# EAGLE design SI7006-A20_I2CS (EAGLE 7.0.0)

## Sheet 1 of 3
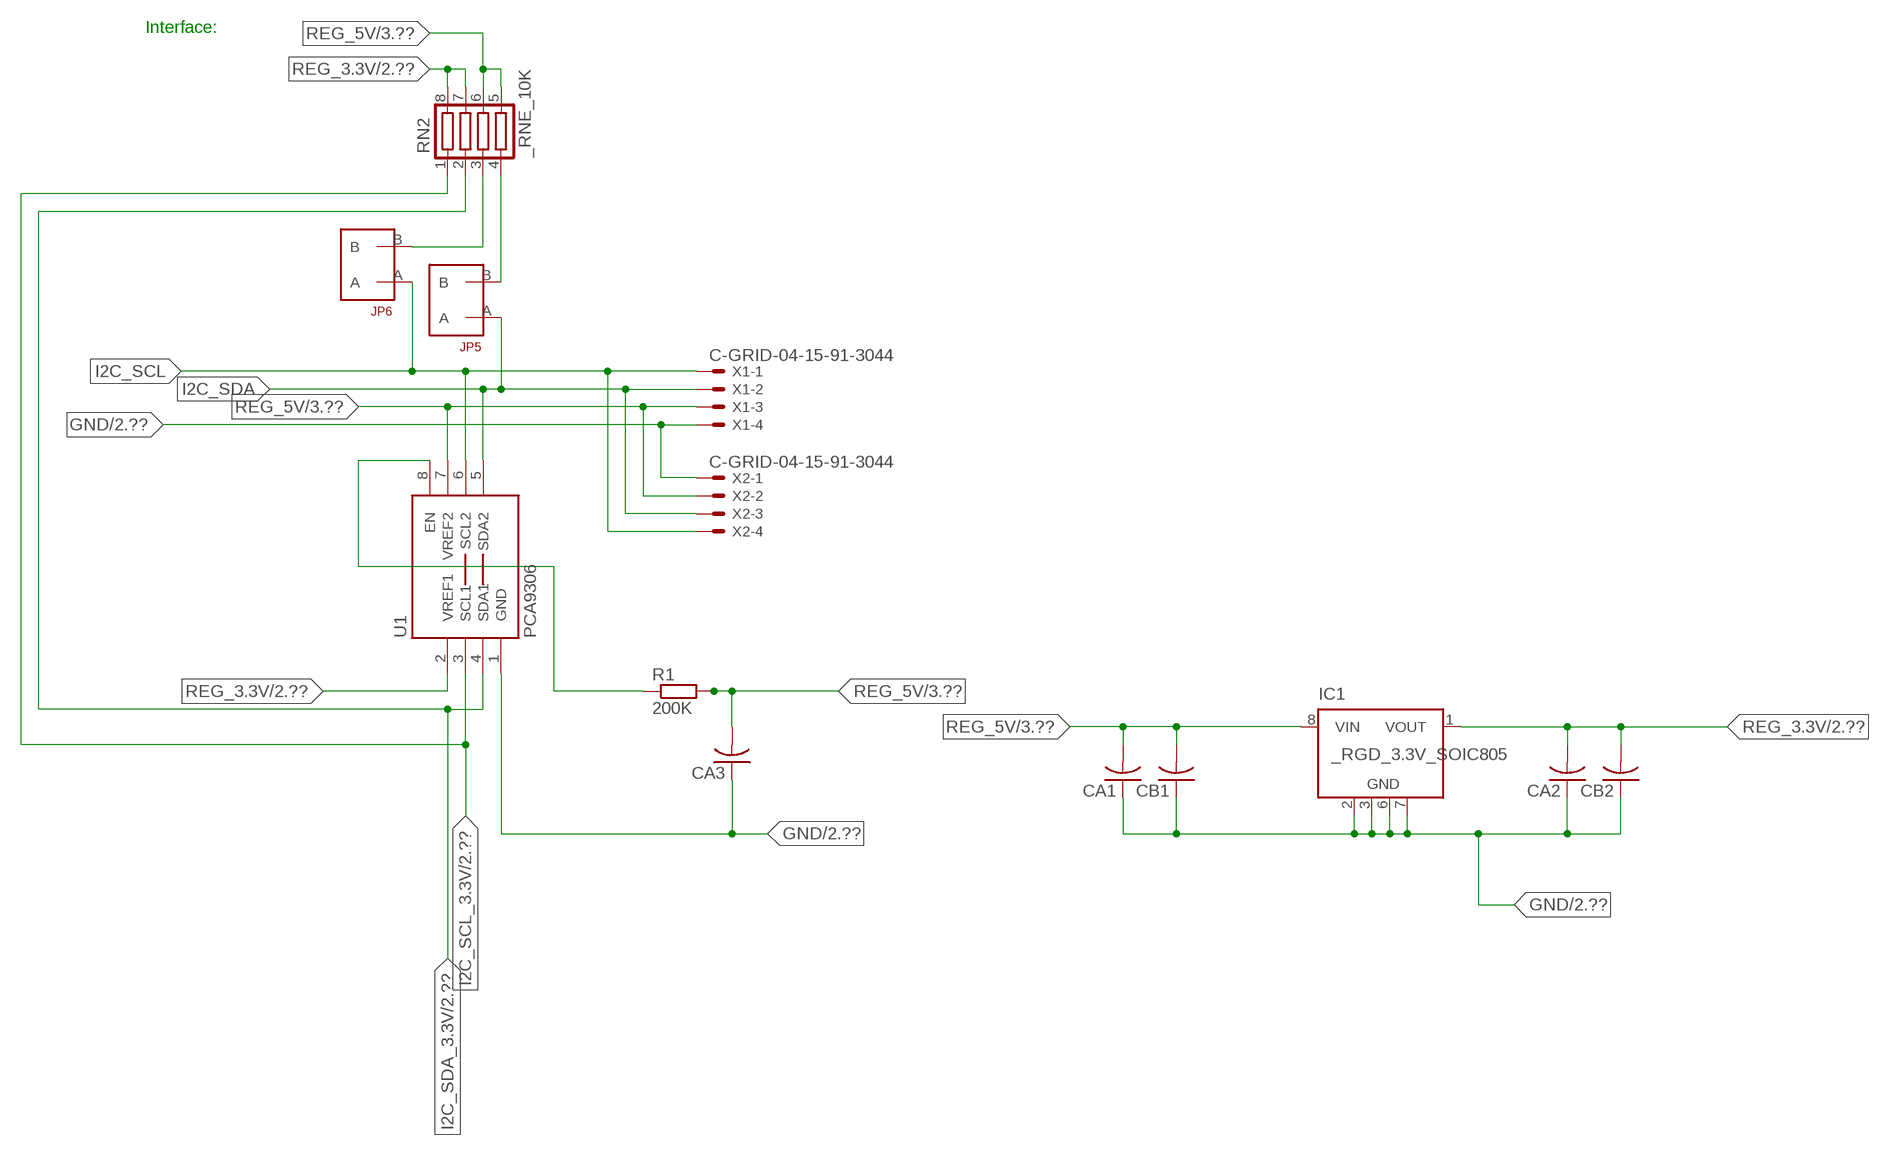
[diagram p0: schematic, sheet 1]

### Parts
CA1  CC1206KRX7R9BB104  [.1UF]
CA2  CC1206KRX7R9BB104  [.1UF]
CA3  CC1206KRX7R9BB104  [.1UF]
CB1  TMK316F106ZL-TC1206K  [TMK316F106ZL-T]
CB2  TMK316F106ZL-TC1206K  [TMK316F106ZL-T]
IC1  _RGD_3.3V_SOIC805  [_RGC_3.3V_SOIC8]
JP5  JUMPER_1X2_2MM  [JUMPER_1X2_2MM]
JP6  JUMPER_1X2_2MM  [JUMPER_1X2_2MM]
R1  200K  RESISTOR_SMT-0603  [R603]
RN2  _RNE_10K  [RNE]
U1  PCA9306  PCA9306_NCD  [PSOP-8]
X1  C-GRID-04-15-91-3044  [15-91-04]
X2  C-GRID-04-15-91-3044  [15-91-04]

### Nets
GND: CA1.1 CA2.1 CA3.1 CB1.1 CB2.1 IC1.2(GND) IC1.3(GND) IC1.6(GND) IC1.7(GND) U1.1(GND) X1.4 X2.1 ; also sheet 2,3
I2C_SCL: JP6.A U1.6(SCL2) X1.1 X2.4
I2C_SCL_3.3V: RN2.1 U1.3(SCL1) ; also sheet 2
I2C_SDA: JP5.A U1.5(SDA2) X1.2 X2.3
I2C_SDA_3.3V: RN2.2 U1.4(SDA1) ; also sheet 2
N$1: JP6.B RN2.3
N$2: JP5.B RN2.4
N$3: R1.1 U1.8(EN)
REG_3.3V: CA2.2 CB2.2 IC1.1(VOUT) RN2.7 RN2.8 U1.2(VREF1) ; also sheet 2
REG_5V: CA1.2 CA3.2 CB1.2 IC1.8(VIN) R1.2 RN2.5 RN2.6 U1.7(VREF2) X1.3 X2.2 ; also sheet 3
Unconnected: IC1.4(NC) IC1.5(NC)

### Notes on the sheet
- Interface:

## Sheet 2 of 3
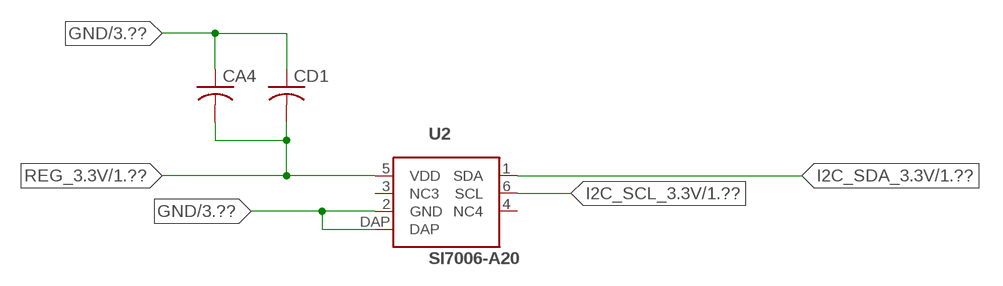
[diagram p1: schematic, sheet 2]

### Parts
CA4  _CA_.10UF_50VC1206K  [_CA_.1UF_50V]
CD1  _CD_10NF_50VC1206K  [_CD_10NF_50V]
U2  SI7006-A20  SI7020-A10  [DFN6]

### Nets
GND: CA4.1 CD1.1 U2.2(GND) U2.DAP ; also sheet 1,3
I2C_SCL_3.3V: U2.6(SCL) ; also sheet 1
I2C_SDA_3.3V: U2.1(SDA) ; also sheet 1
REG_3.3V: CA4.2 CD1.2 U2.5(VDD) ; also sheet 1
Unconnected: U2.3(NC3) U2.4(NC4)

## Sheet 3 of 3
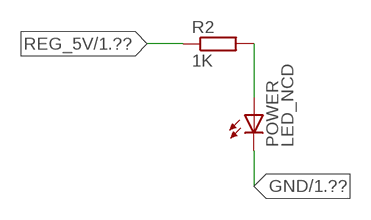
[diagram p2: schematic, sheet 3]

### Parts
POWER  LED_NCD  [CHIPLED_0603]
R2  1K  RESISTOR_SMT-0402  [R402]

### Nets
GND: POWER.C ; also sheet 1,2
N$4: POWER.A R2.2
REG_5V: R2.1 ; also sheet 1

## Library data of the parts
CA1-CA3 = NCD_ULTIMATE_LIBRARY:CC1206KRX7R9BB104: Capacitor CA .1uF 50V SMT C1206K CC1206KRX7R9BB104
CA4 = NCD_ULTIMATE_LIBRARY:_CA_.10UF_50V: Capacitor .1uF SMT
CB1 CB2 = NCD_ULTIMATE_LIBRARY:TMK316F106ZL-T: Capacitor CB 10uF SMT 1206 TMK316F106ZL-T
CD1 = NCD_ULTIMATE_LIBRARY:_CD_10NF_50V: Capacitor 10nF SMT
IC1 = NCD_ULTIMATE_LIBRARY:_RGD_3.3V_SOIC8: Regulator Linear 3.3V Chip Positive VOLTAGE REGULATOR Digikey 497-1199-2-ND/L78L33ACD13TR
JP5 JP6 = NCD_ULTIMATE_CONNECTORS:JUMPER_1X2_2MM
POWER = NCD_ULTIMATE_LIBRARY:LED_NCD: LED Digikey 754-1132-2-ND/APT2012SRCPRV
R1 R2 = NCD_ULTIMATE_LIBRARY:RESISTOR_SMT: NCD Resistor
RN2 = NCD_ULTIMATE_LIBRARY:_RNE_10K: Resistor Array RNE SMT 10K x 4 Single Resistor Source: http://www.ctscorp.com/components/Datasheets/CTSChipArrayDs.pdf Digikey 742C083103JPTR-ND/742C083103JP; OC_FARNELL: unknown; OC_NEWARK: unknown
U1 = NCD_ULTIMATE_LIBRARY:PCA9306_NCD: NCD Bidirectional I2C level shifter. NOT compatible with all available part number pinout schemes- DOUBLE CHECK!!!; PROD_ID: IC-10023
U2 = NCD_ULTIMATE_bhaskar:SI7020
X1 X2 = NCD_ULTIMATE_CONNECTORS:C-GRID-04: CONNECTOR 4-Pos I2C wire to board 2.54 mm (0.100") pitch header Digikey WM1342-ND/0015912045; OC_FARNELL: unknown; OC_NEWARK: unknown

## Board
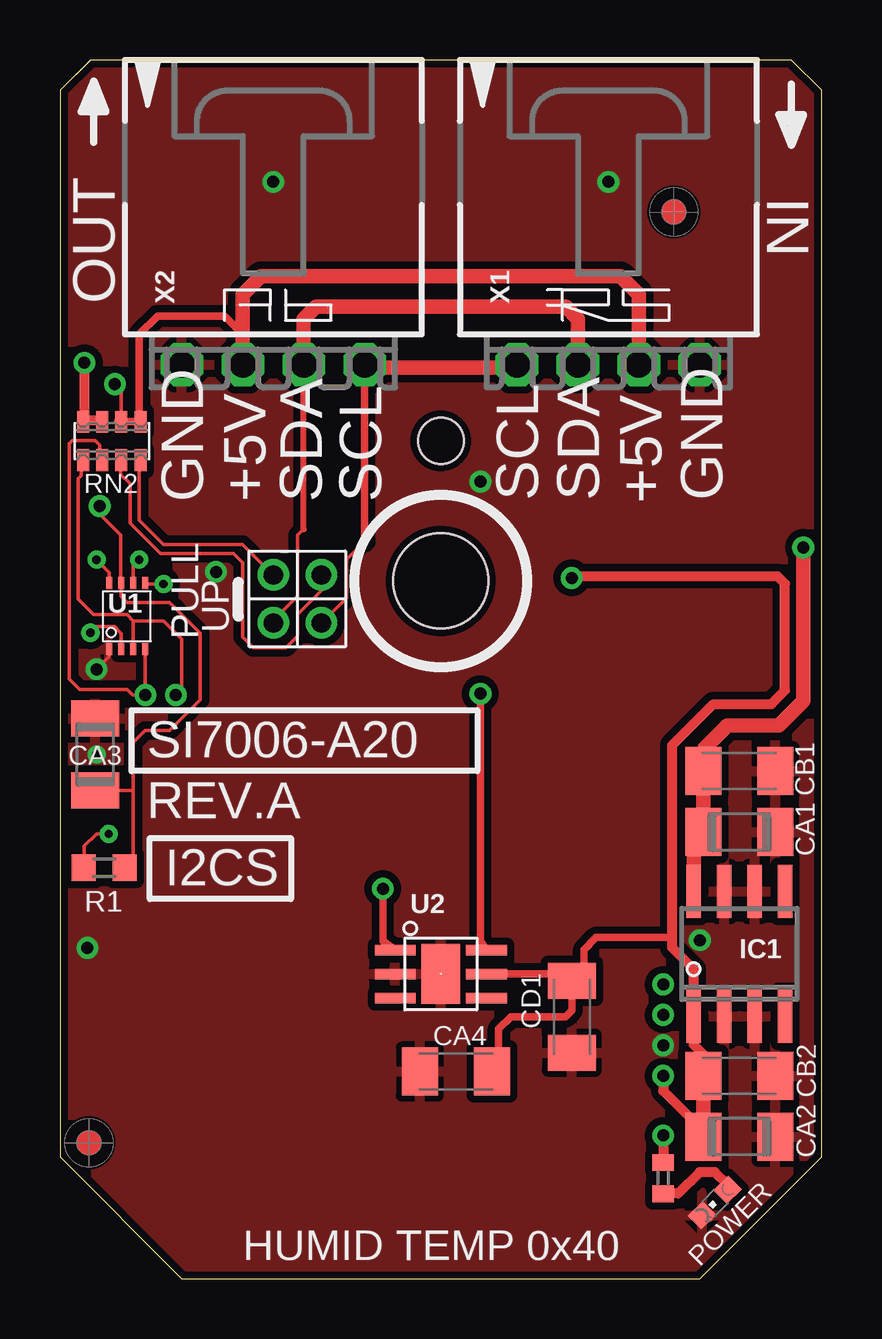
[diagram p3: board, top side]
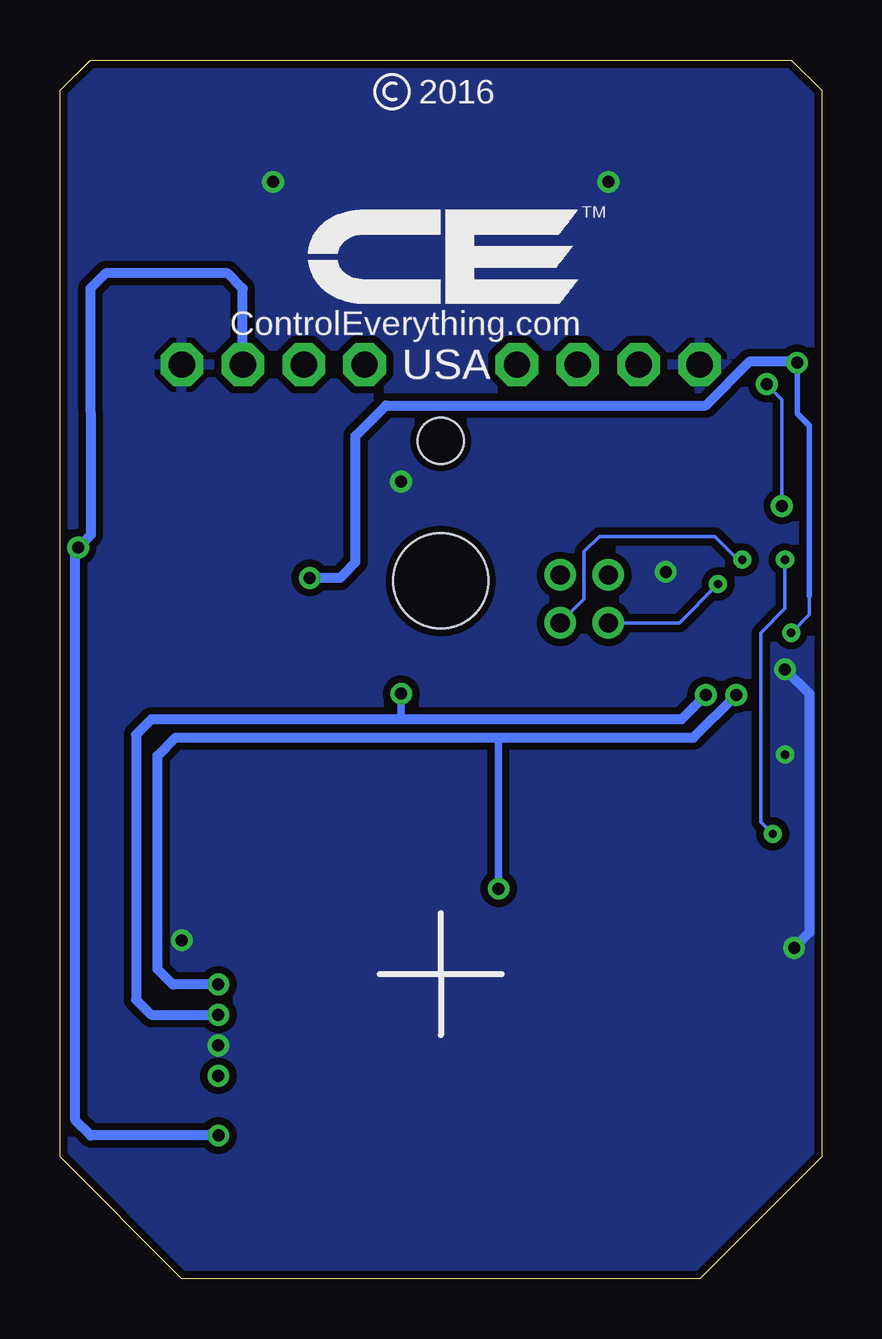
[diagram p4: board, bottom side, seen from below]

Size 31.75 x 50.8 mm. Coordinates in mm from the lower left corner, seen from the top.
Outline: 48 segments
Copper layers (1*16): Top 0.035mm / dielectric 1.5mm / Bottom 0.035mm
Design rules "default": minimum track width 5mil, minimum drill 24mil, track to track 5mil, track to pad 5mil, pad to pad 5mil, via to via 5mil, smd to smd 5mil, copper to edge 10mil, drill to drill 8mil, minimum pad ring 10mil, minimum via ring 8mil, stop-mask expansion 2mil, vias tented up to drill 0mil, thermal gap 10mil
Holes 3.96 mm at 15.88,29.08
Holes 1.91 mm at 15.88,34.93

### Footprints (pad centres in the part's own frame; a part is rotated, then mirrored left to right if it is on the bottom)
.1UF = smd 1.5 x 2: 1 -1.5,0; 2 1.5,0
_CA_.1UF_50V = smd 1.5 x 2: 1 -1.5,0; 2 1.5,0
TMK316F106ZL-T = smd 1.5 x 2: 1 -1.5,0; 2 1.5,0
_CD_10NF_50V = smd 1.5 x 2: 1 -1.5,0; 2 1.5,0
_RGC_3.3V_SOIC8 = smd 0.6 x 2.2: 1 -1.905,-2.6; 2 -0.635,-2.6; 3 0.635,-2.6; 4 1.905,-2.6; 5 1.905,2.6; 6 0.635,2.6; 7 -0.635,2.6; 8 -1.905,2.6
JUMPER_1X2_2MM = drill 0.8: A 0,2; B 0,0
CHIPLED_0603 = smd 0.8 x 0.876: A 0,-0.75; C 0,0.75
R603 = smd 1 x 1.1: 1 -0.85,0; 2 0.85,0
R402 = smd 0.7 x 0.9: 1 -0.65,0; 2 0.65,0
RNE = smd 0.5 x 0.9: 1 -1.2,-0.8; 2 -0.4,-0.8; 3 0.4,-0.8; 4 1.2,-0.8; 5 1.2,0.8; 6 0.4,0.8; 7 -0.4,0.8; 8 -1.2,0.8
PSOP-8 = smd 0.25 x 0.5: 1 -0.73,-1.37; 2 -0.23,-1.37; 3 0.27,-1.37; 4 0.77,-1.37; 5 0.77,1.38; 6 0.27,1.38; 7 -0.23,1.38; 8 -0.73,1.38
DFN6 = smd 1.7 x 0.45: 1 -1.9,1; 2 -1.9,0; 3 -1.9,-1; 4 1.9,-1; 5 1.9,0; 6 1.9,1 | smd 1.6 x 2.5: DAP 0,0
15-91-04 = drill 1.1 pad 1.778 octagon: 1 -3.81,-7.62; 2 -1.27,-7.62; 3 1.27,-7.62; 4 3.81,-7.62

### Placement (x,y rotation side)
CA1  28.32,18.62 180 top
CA2  28.32,5.92 180 top
CA3  1.46,21.86 270 top
CA4  16.51,8.64 0 top
CB1  28.32,21.16 180 top
CB2  28.32,8.46 180 top
CD1  21.34,10.92 90 top
IC1  28.32,13.54 0 top
JP5  8.89,29.34 180 top
JP6  10.9,29.34 180 top
POWER  27.3,3.18 135 top
R1  1.84,17.13 0 top
R2  25.15,4.19 270 top
RN2  2.16,34.93 0 top
U1  2.79,27.61 0 top
U2  15.88,12.7 0 top
U$5  [VISION_REF10]  1.21,5.66 90 top
U$28  [VISION_REF10]  25.59,44.46 90 top
X1  22.86,45.72 0 top
X2  8.89,45.72 0 top

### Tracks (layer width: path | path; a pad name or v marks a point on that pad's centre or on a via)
GND  (via drill 0.35, 0.5)
  Top 0.152: CA3.1 1.52,23.42 1.52,23.62 | v1.52,25.4 2.06,25.94 U1.1
  Bottom 0.406: v1.52,25.4 0.51,24.38 0.51,14.43 v1.15,13.79
  other vias: 8.89,45.72 22.86,45.72 25.15,9.73 17.53,33.22 26.67,14.11 6.5,29.46 1.52,21.84
  pour Bottom (isolate 0.305): -0.64,5.08 -0.64,49.53 1.27,51.44 30.48,51.44 32.38,49.53 32.38,5.08 26.67,-0.63 5.08,-0.63
  pour Top (isolate 0.305): 4.45,-1.27 -1.27,4.45 -1.27,50.17 0.64,52.07 31.11,52.07 33.02,50.17 33.02,4.45 27.3,-1.27
I2C_SCL  (via drill 0.35)
  Top 0.152: 12.7,30.73 11.94,29.97 11.94,28.38 JP6.A | v3.3,29.97 3.06,29.73 U1.6
  Top 0.305: 12.7,30.73 X2.4
  Top 0.406: X2.4 12.7,37.97 | 19.05,37.97 X1.1
  Top 0.61: 12.7,37.97 19.05,37.97
  Bottom 0.152: JP6.A 9.91,28.33 9.91,30.3 9.27,30.94 4.45,30.94 3.48,29.97 v3.3,29.97
I2C_SCL_3.3V  (via drill 0.5)
  Top 0.152: RN2.1 0.89,34.07 0.89,33.48 0.77,33.35 0.77,28.33 1.41,27.69 2.79,27.69 3.06,27.42 | 3.06,27.42 U1.3 | v4.83,24.33 5.08,24.59 5.08,26.67 4.33,27.42 3.06,27.42
  Top 0.305: U2.6 17.53,14.09 v17.53,24.38
  Bottom 0.305: v17.53,24.38 17.53,23.32
  Bottom 0.406: v4.83,24.33 5.84,23.32 17.53,23.32 27.94,23.32 28.58,22.68 28.58,11.63 27.94,11 v25.15,11
I2C_SDA  (via drill 0.35)
  Top 0.152: JP5.A 8.89,27.44 9.91,28.45 9.91,30.99 10.16,31.24 | U1.5 3.6,28.96 v4.32,28.96
  Top 0.254: 10.16,31.24 10.16,31.25 X2.3
  Top 0.61: X2.3 10.16,40.01 10.67,40.51 21.09,40.51 21.59,40.01 X1.2
  Bottom 0.152: v4.32,28.96 5.94,27.34 JP5.A
I2C_SDA_3.3V  (via drill 0.5)
  Top 0.152: RN2.2 1.65,34.14 1.65,34.75 1.46,34.94 0.51,34.94 0.38,34.81 0.38,26.37 0.38,26.36 0.38,24.99 0.81,24.56 2.79,24.56 3.02,24.33 v3.56,24.33 v3.56,24.34 U1.4
  Top 0.305: U2.1 13.46,14.09 v13.46,16.26
  Bottom 0.305: v13.46,16.26 13.46,22.56
  Bottom 0.406: v25.15,12.27 27.05,12.27 27.69,12.9 27.69,21.79 26.93,22.56 13.46,22.56 5.34,22.56 v3.56,24.33
N$1
  Top 0.152: JP6.B 10.92,29.31 10.92,28.7 9.91,27.69 9.91,26.8 9.42,26.31 8.06,26.31 7.62,26.75 7.62,29.84 7.24,30.23 4.19,30.23 2.92,31.5 2.92,33.15 2.54,33.53 2.54,34.1 RN2.3
  Top 0.305: 2.54,34.02 RN2.3
N$2
  Top 0.152: JP5.B 7.62,30.61 4.32,30.61 3.3,31.62 3.3,34.07 RN2.4
  Top 0.305: 3.37,33.88 RN2.4
N$3  (via drill 0.35)
  Top 0.152: R1.1 1.02,17.16 1.02,18.03 1.52,18.54 v2.03,18.54 | v1.52,29.97 2.06,29.44 U1.8
  Bottom 0.152: v2.03,18.54 2.54,19.05 2.54,26.92 1.52,27.94 v1.52,29.97
N$4
  Top 0.406: POWER.A 27.84,3.92 27.3,4.45 26.67,4.45 25.78,3.56 25.16,3.56 R2.2
REG_3.3V  (via drill 0.35, 0.5)
  Top 0.152: v1.27,26.92 1.52,27.18 2.29,27.18 2.56,26.9 U1.2
  Top 0.305: CA4.2 18.29,9.42 18.29,10.41 18.8,10.92 21.08,10.92 21.34,11.18 CD1.2 | CD1.2 21.84,12.93 21.84,13.72 22.35,14.22 25.53,14.22 | U2.5 21.34,12.7 CD1.2
  Top 0.406: CB2.2 26.82,9.35 26.42,9.75 26.42,10.36 | v25.15,8.46 25.15,7.82 26.42,6.55 26.82,6.55 | IC1.1 26.42,12.9 25.53,13.79 25.53,14.22 25.53,22.24 27.24,23.95 29.66,23.95 30.23,24.52 30.23,28.97 29.91,29.29 21.41,29.29 v21.34,29.21 | 26.52,5.62 CA2.2 | v1.02,38.18 1.02,35.78 | 1.02,35.78 RN2.8 | 1.02,35.78 1.71,35.78 RN2.7
  Top 0.61: CB2.2 26.82,6.55 CA2.2 | 26.42,10.36 IC1.1
  Bottom 0.152: 0.51,28.45 0.51,27.69 v1.27,26.92
  Bottom 0.229: 0.51,28.45 0.51,35.56 1.02,36.07 v1.02,38.18
  Bottom 0.406: v1.02,38.18 1.08,38.24 2.99,38.24 4.83,36.4 18.16,36.4 19.43,35.13 19.43,29.87 19.94,29.34 20.07,29.21 v21.34,29.21
REG_5V  (via drill 0.5)
  Top 0.152: RN2.6 2.56,37.01 v2.29,37.29 | R1.2 3.05,17.49 3.05,20.36 | 3.05,20.36 3.05,22.35 3.56,22.86 4.57,22.86 5.84,24.13 5.84,26.92 4.57,28.19 2.79,28.19 2.56,28.43 U1.7 2.54,29.01 2.54,30.99 1.65,31.87 v1.65,32.21 | CA3.2 3.05,20.36
  Top 0.305: 7.62,39.37 7.5,39.37 | 2.42,35.74 RN2.6 RN2.5 3.31,35.8 3.31,39.37 4.07,40.13 6.86,40.13 7.62,39.37 | X2.2 7.62,39.37
  Top 0.406: v25.15,5.97 R2.1
  Top 0.61: X1.3 24.13,41.02 23.37,41.78 8.38,41.78 7.62,41.02 X2.2 | IC1.8 26.42,18.21 CA1.2 CB1.2 26.86,21.2 26.86,22.11 27.82,23.06 29.98,23.06 30.99,24.08 v30.99,30.48
  Bottom 0.152: v1.65,32.21 1.65,36.65 v2.29,37.29
  Bottom 0.406: X1.3 24.13,41.28 24.77,41.91 29.84,41.91 30.48,41.27 30.47,31 v30.99,30.48 31.11,30.36 31.11,6.6 30.48,5.97 v25.15,5.97

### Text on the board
tNames: IN | OUT | GND | +5V | SDA | SCL | SCL | SDA | +5V | GND | PULL | UP | SI7006-A20 | REV.A | I2CS | HUMID TEMP 0x40
bNames: 2016 | TM | ControlEverything.com | USA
